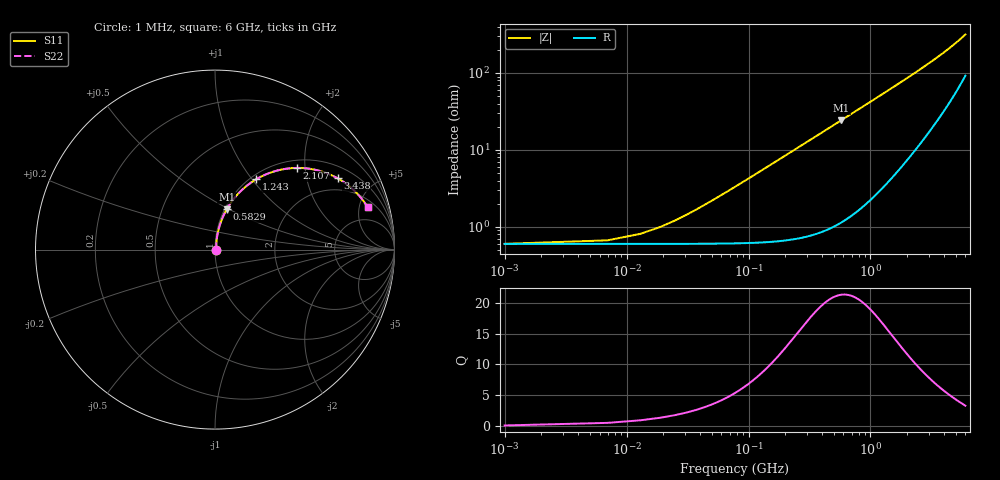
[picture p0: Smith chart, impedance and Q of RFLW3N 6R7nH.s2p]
!Vishay Electro-Films
!RFLW3N6700C - 6.7 nH Spiral Inductor on Quartz
!Measured in series configuration
!May 2011
# GHz S MA R 50
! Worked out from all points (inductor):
!   1001 points, 1 MHz to 6 GHz, reference 50 ohm
!   read as one part in series: L = 6.69 nH near 48.99 MHz
!   highest Q = 21.3 at 576.9 MHz (marker M1), where L = 6.7 nH
!   S11 on the Smith chart (normalised r, x): 1 MHz: 1.01, +0.00; 582.9 MHz: 1.02, +0.49; 1.243 GHz: 1.06, +1.05; 2.107 GHz: 1.16, +1.81; 3.438 GHz: 1.45, +3.07; 6 GHz: 2.85, +6.07
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0.001  0.005976 4.0  0.994 -0.0  0.994 -0.0  0.005976 4.0
0.018997  0.009932 52.6  0.994 -0.5  0.994 -0.5  0.009932 52.6
0.054991  0.02375 74.0  0.9937 -1.3  0.9937 -1.3  0.02375 74.0
0.078987  0.03355 77.7  0.9934 -1.9  0.9934 -1.9  0.03355 77.7
0.12098  0.05088 80.1  0.9925 -2.9  0.9925 -2.9  0.05088 80.1
0.168972  0.07072 80.8  0.9911 -4.0  0.9911 -4.0  0.07072 80.8
0.24096  0.1004 80.3  0.9881 -5.7  0.9881 -5.7  0.1004 80.3
0.330945  0.1371 78.9  0.983 -7.9  0.983 -7.9  0.1371 78.9
0.444926  0.1827 76.7  0.9742 -10.5  0.9742 -10.5  0.1827 76.7
0.576904  0.2339 73.8  0.9614 -13.5  0.9614 -13.5  0.2339 73.8
0.582903  0.2362 73.7  0.9607 -13.6  0.9607 -13.6  0.2362 73.7
0.774871  0.3067 69.4  0.9372 -17.8  0.9372 -17.8  0.3067 69.4
1.00283  0.3835 64.5  0.9035 -22.5  0.9035 -22.5  0.3835 64.5
1.24279  0.4557 59.5  0.8634 -27.1  0.8634 -27.1  0.4557 59.5
1.60273  0.5471 52.8  0.799 -33.1  0.799 -33.1  0.5471 52.8
2.00467  0.6276 46.4  0.7266 -38.7  0.7266 -38.7  0.6276 46.4
2.10665  0.6449 44.9  0.7086 -40.0  0.7086 -40.0  0.6449 44.9
3.0005  0.7554 34.2  0.5669 -48.5  0.5669 -48.5  0.7554 34.2
3.43843  0.7901 30.2  0.5086 -51.4  0.5086 -51.4  0.7901 30.2
4.00233  0.823 25.9  0.4434 -54.2  0.4434 -54.2  0.823 25.9
5.00417  0.8607 19.9  0.35 -57.0  0.35 -57.0  0.8607 19.9
6  0.8828 15.4  0.2784 -57.6  0.2784 -57.6  0.8828 15.4
